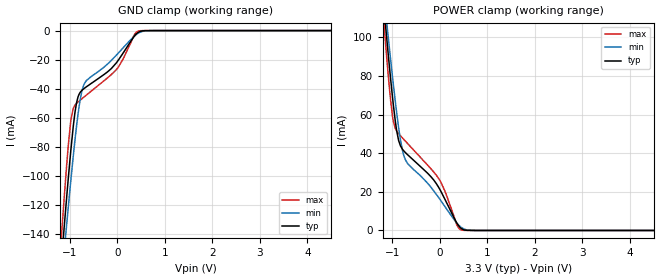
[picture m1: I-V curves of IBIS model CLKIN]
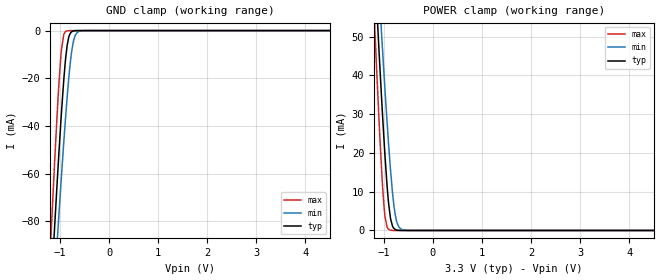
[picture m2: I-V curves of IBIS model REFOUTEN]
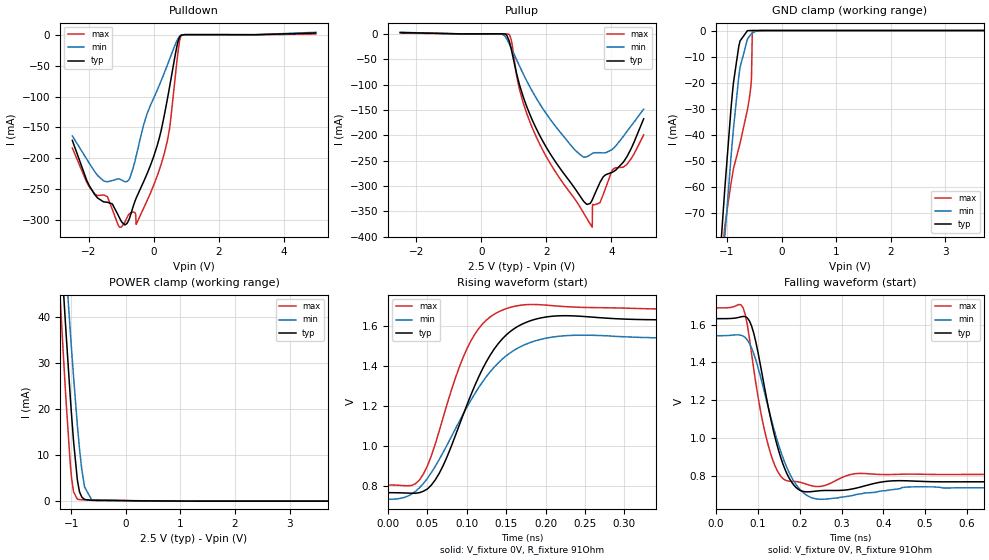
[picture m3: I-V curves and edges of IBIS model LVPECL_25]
| Texas Instruments Incorporated
| 3-GHz, 8-Output Differential Fanout Buffer / Level Translator
| Marketing part#   Voltage Range   Package-type   #pins/pkg drawing
| LMK00338   3.15V - 3.45V   LLP   40-pin SQ
[IBIS Ver]   4.1
[File name]   lmk00338.ibs
[File Rev]   1.1
[Date]   1/27/2014
[Source]   Model built from spectre simulations at:
   Texas Instruments Incorporated.
   Analog-eLab, HPA
   12500 TI Blvd
   Dallas, TX -75243
   For Support e-mail: elab_ibis@list.ti.com
[Notes]   Revision History
   Rev 1.1: 1/27/2014
   - Correct pin names/assignments for Pins 11, 19 and 32
   Rev 1.0: 3/12/2012
   - ccomp values are based on PVT settings:
   WEAK: Low Voltage, High Temperature, Weak Process
   NOM: Nominal Voltage, Nominal Temperature, Nominal Process
   STRONG: High Voltage, Low Temperature, Fast Process
   - User may change ccomp in the order of number values as
   per end simulator used
   - C_comp although listed in numberical order of value are obtained from varying PVT conditions.
   For PVT conditions for eachspecific value, refer to the buffer description under repective [Model].
   IBIS model user is responsible for using appropriate C_comp to simulate for Signal Integrity.
   - LVPECL Simulation recommendation:
   Use low value (1nF or less) for AC coupling.
   Larger values will result in long settling times.
   -PullUp and Pulldown non-monotonic for LVPECL and REFOUT models
[Disclaimer]  This model is designed as an aid for customers of Texas Instruments
 TI and its licensors and suppliers make no warranties, either expressed
 or implied, with respect to this  model, including the warranties of
 merchantability or fitness for a particular purpose.
 The model is provided solely on an "as is" basis. The entire risk as to
 its quality and performance is with the customer.
[Copyright] (C)Copyright 2012 Texas Instruments Incorporated.
   All rights reserved.
[Component]   LMK00308SQ
[Manufacturer]  Texas Instruments Incorporated
[Package]   |40-pin LLP SQ package
|   typ   min   max
R_pkg   0   0   0
L_pkg   0   0   0
C_pkg   0   0   0
[Pin]   signal_name   model_name   R_pin   L_pin   C_pin
1   CLKoutA0   DIFFOUT
2   CLKoutA0*   DIFFOUT
3   VCC0A   POWER
4   CLKoutA1   DIFFOUT
5   CLKoutA1*   DIFFOUT
6   VCC0A   POWER
7   CLKoutA2   DIFFOUT
8   CLKoutA2*   DIFFOUT
9   CLKout32   DIFFOUT
10   CLKout32*   DIFFOUT
11   CLKoutA_EN   REFOUTEN
12   VCC   POWER
13   OSCin   NC
14   OSCout   NC
15   CLKin_SEL0   NC
16   CLKin0   CLKIN
17   CLKin0*   CLKIN
18   CLKin_SEL1   NC
19   CLKoutB_EN   REFOUTEN
20   GND   GND
21   CLKoutB3*   DIFFOUT
22   CLKoutB3   DIFFOUT
23   CLKoutB2*   DIFFOUT
24   CLKoutB2   DIFFOUT
25   VCC0B   POWER
26   CLKoutB1*   DIFFOUT
27   CLKoutB1   DIFFOUT
28   VCC0B   POWER
29   CLKoutB0*   DIFFOUT
30   CLKoutB0   DIFFOUT
31   GND   GND
32   VCC   POWER
33   CLKin1*   CLKIN
34   CLKin1   CLKIN
35   VCC   POWER
36   REFout   REFOUT
37   VCC0C   POWER
38   REFout_EN   REFOUTEN
39   CLKoutA_TYPE1   NC
40   GND   GND
41   DAP   NC
[Diff pin]  inv_pin  vdiff  tdelay_typ  tdelay_min  tdelay_max
 3   4   NA   0.0s   0.0s   0.0s
 6   7   NA   0.0s   0.0s   0.0s
 8   9   NA   0.0s   0.0s   0.0s
20   21   NA   0.0s   0.0s   0.0s
22   23   NA   0.0s   0.0s   0.0s
25   26   NA   0.0s   0.0s   0.0s
15   16   0.15   NA  NA  NA   | Diff-in
31   30   0.15   NA  NA  NA   | Diff-in
| Model REFOUT
[Model Selector]   REFOUT
REFOUT_33   3.3 volt Vcc
REFOUT_25   2.5 volt Vcc
| Model DIFFOUT
[Model Selector]   DIFFOUT
LVPECL_33   3.3 volt Vcc
LVPECL_25   2.5 volt Vcc
LVDS_33   3.3 volt Vcc
LVDS_25   2.5 volt Vcc
HCSL_33   3.3 volt Vcc
HCSL_25   2.5 volt Vcc
[Define Package Model]  llp40_lmk00308
[Manufacturer]  Unknown
[OEM]  Unknown
[Description]  ]  Evaled at 2GHz using Buildsheet AD#LMK00308SQ-01 RevA
[Number Of Pins]  41
[Pin Numbers]
|Pin Num   Terminal Name
1   | L1:1
2   | L2:2
3   | L3:3
4   | L4:4
5   | L5:5
6   | L6:6
7   | L7:7
8   | L8:8
9   | L9:9
10   | L10:10
11   | L11:11
12   | L12:12
13   | L13:13
14   | L14:14
15   | L15:15
16   | L16:16
17   | L17:17
18   | L18:18
19   | L19:19
20   | L20:20
21   | L21:21
22   | L22:22
23   | L23:23
24   | L24:24
25   | L25:25
26   | L26:26
27   | L27:27
28   | L28:28
29   | L29:29
30   | L30:30
31   | L31:31
32   | L32:32
33   | L33:33
34   | L34:34
35   | L35:35
36   | L36:36
37   | L37:37
38   | L38:38
39   | L39:39
40   | L40:40
41   | LDAP:41
[Model Data]
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[End Model Data]
[End Package Model]
| Models and submodels in the file (10): CLKIN (Input), REFOUTEN (Input), LVPECL_25 (3-state), LVPECL_33 (3-state), LVDS_25 (Output), LVDS_33 (Output), HCSL_25 (Open_source), HCSL_33 (Open_source), REFOUT_25 (Output), REFOUT_33 (Output)
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|   Model   CLKIN
[Model]   CLKIN
Model_type   Input
Vinl = 1.2
Vinh = 1.35
|   typ   min   max
C_comp   0.334pF   0.334pF   0.334pF
[Voltage Range]   3.3   3.125   3.465
[Temperature Range]   45   125   -40
[Power Clamp Reference]   3.3   3.125   3.465
[GND Clamp Reference]   0   0   0
[GND Clamp]
|   Voltage   I(typ)   I(min)   I(max)
-3.3V     -1.09A     -1.005A    -1.209A
-1.181V   -161.9mA   -176mA     -145.1mA
-1.112V   -133.8mA   -150.7mA   -113.6mA
-1.063V   -114.4mA   -133.1mA   -92.33mA
-973.5mV  -81.6mA    -102.3mA   -61.43mA
-924mV    -65.73mA   -86.12mA   -53.42mA
-854.7mV  -49.53mA   -65.42mA   -49.97mA
-775.5mV  -42.3mA    -46.78mA   -47.7mA
-706.2mV  -40.03mA   -37.67mA   -45.84mA
-3.3mV    -21.51mA   -16.37mA   -26.2mA
432.3mV   -1.452mA   -2.001mA   -480.3uA
6.59V     0A         0A         0A
[POWER Clamp]
|   Voltage   I(typ)   I(min)   I(max)
-3.3V     736.4mA    674.5mA    821.9mA
-1.181V   117.5mA    123.8mA    109.8mA
-1.112V   98.9mA     107.1mA    88.87mA
-1.033V   78.62mA    88.59mA    67.5mA
-973.5mV  64.71mA    75.26mA    56.32mA
-914.1mV  53.13mA    62.75mA    51.87mA
-864.6mV  46.64mA    53.33mA    50.15mA
-745.8mV  40.96mA    38.12mA    46.9mA
-13.2mV   21.94mA    16.71mA    26.59mA
353.1mV   4.136mA    4.038mA    3.278mA
442.2mV   1.233mA    1.8mA      362.3uA
6.59V     0A         0A         0A
|   Model REFOUTEN
[Model]   REFOUTEN
Model_type   Input
Vinl = 0.8
Vinh = 2.0
|   typ   min   max
C_comp   0.3093pF   0.3093pF   0.3093pF
[Voltage Range]   3.3   3.125   3.465
[Temperature Range]   45   125   -40
[Power Clamp Reference]   3.3   3.125   3.465
[GND Clamp Reference]   0   0   0
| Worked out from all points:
|   GND clamp passes 1 mA (typ) near -0.79 V on its own axis
|   POWER clamp passes 1 mA (typ) near -0.82 V on its own axis
[GND Clamp]
|   Voltage   I(typ)   I(min)   I(max)
-3.3V     -965.6mA   -893.6mA   -1.069A
-1.181V   -108.3mA   -129.3mA   -84.35mA
-1.112V   -82.59mA   -106mA     -55.39mA
-1.043V   -57.82mA   -83.32mA   -28.72mA
-973.5mV  -34.81mA   -61.42mA   -8.124mA
-924mV    -20.4mA    -46.56mA   -1.597mA
-884.4mV  -11.09mA   -35.36mA   -347uA
-825mV    -2.889mA   -20.4mA    -26.1uA
-745.8mV  -310.8uA   -6.404mA   -528.4nA
-676.5mV  -33.31uA   -1.499mA   -14.52nA
-577.5mV  -943.1nA   -148.2uA   0A
6.59V     0A         0A         0A
[POWER Clamp]
|   Voltage   I(typ)   I(min)   I(max)
-3.3V     638.8mA    590.5mA    708.3mA
-1.191V   69.15mA    82.63mA    53.96mA
-1.181V   66.68mA    80.4mA     51.15mA
-1.102V   47.28mA    62.82mA    29.5mA
-1.033V   31.21mA    47.91mA    12.87mA
-993.3mV  22.67mA    39.68mA    5.73mA
-933.9mV  11.5mA     27.94mA    888.7uA
-864.6mV  3.112mA    15.73mA    67.37uA
-805.2mV  711.5uA    7.563mA    4.089uA
-745.8mV  145.3uA    2.701mA    212.4nA
-577.5mV  412.5nA    72uA       0A
6.59V     0A         0A         0A
|   Model LVPECL_25
[Model]   LVPECL_25
Model_type   3-state
Polarity   Non-Inverting
Rref =   91.0000
Vmeas =   1.99
|   typ   min   max
|   Nom   Strong   Weak
C_comp   2.0749pF   1.9512pF   2.2734pF
|Output in low   Nom   Strong   Weak
|C_Comp   2.0749pF   1.9512pF   2.2734pF
|Output in High   Nom   Strong   Weak
|C_Comp   0.7651pF   0.6976pF   0.7651pF
[Voltage Range]   2.5   2.375   2.625
[Temperature Range]   45   125   -40
[Pullup Reference]   2.5   2.375   2.625
[Pulldown Reference]   -0   0   -0
[Power Clamp Reference]   2.5   2.375   2.625
[GND Clamp Reference]   0   -0   -0
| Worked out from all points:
|   slope of the pulldown table from 0 to 0.375 V, typ, clamps not added: 4.73 ohm
|   GND clamp passes 1 mA (typ) near -0.66 V on its own axis
|   POWER clamp passes 1 mA (typ) near -0.81 V on its own axis
|   falling waveform, V_fixture 0V, R_fixture 91Ohm: 20-80 % time 48.8ps typ, 60.3ps min, 41.4ps max; typ from 1.63 V to 0.768 V
|   rising waveform, V_fixture 0V, R_fixture 91Ohm: 20-80 % time 56ps typ, 71.7ps min, 45.7ps max; typ from 0.768 V to 1.63 V
[Pulldown]
|   Voltage   I(typ)   I(min)   I(max)
-2.5V     -170.9mA   -163.7mA   -183.2mA
-1.817V   -258mA     -220.8mA   -256.9mA
-1.42V    -270.8mA   -237.8mA   -261.8mA
-1.045V   -296.5mA   -233.4mA   -311.1mA
-880mV    -307.5mA   -237.7mA   -302.8mA
-625mV    -277.3mA   -215.2mA   -286.5mA
-535mV    -264.3mA   -196.5mA   -306.6mA
-205mV    -225.5mA   -128.7mA   -269.1mA
245mV     -152.3mA   -73.16mA   -207.5mA
492.5mV   -84.88mA   -39.88mA   -152mA
845mV     -1.078mA   -1.179mA   -2.211mA
4.992V    2.59mA     3.71mA     981.9uA
[GND Clamp]
|   Voltage   I(typ)   I(min)   I(max)
-2.5V     -680.7mA   -652.3mA   -694.7mA
-1.135V   -89.97mA   -107.4mA   -101.7mA
-1.045V   -62.74mA   -81.12mA   -76.76mA
-1.038V   -60.54mA   -78.99mA   -75.08mA
-925mV    -30mA      -48.72mA   -58.7mA
-880mV    -20.04mA   -37.72mA   -53.1mA
-760mV    -4.036mA   -14.22mA   -43.38mA
-625mV    -70.9uA    -3.386mA   -30.51mA
-572.5mV  -12.45uA   -1.77mA    -23.42mA
-550mV    -6.1uA     -1.283mA   -18.23mA
-535mV    -3.82uA    -1.017mA   0A
4.992V    0A         0A         0A
[Pullup]
|   Voltage   I(typ)   I(min)   I(max)
-2.5V     2.519mA    2.915mA    1.456mA
845mV     -12.71mA   -18.28mA   -985.4uA
1.167V    -99.82mA   -63.09mA   -109mA
1.58V     -172.3mA   -115.1mA   -187.8mA
2.84V     -301.8mA   -226.4mA   -322.9mA
3.245V    -336.5mA   -242.4mA   -364.4mA
3.41V     -327.6mA   -236.1mA   -381.3mA
3.417V    -326.6mA   -235.8mA   -336.4mA
3.65V     -292.8mA   -234.5mA   -332.6mA
4.032V    -272.8mA   -227.6mA   -268.4mA
4.475V    -242.6mA   -192.8mA   -257.7mA
4.992V    -167.7mA   -148.6mA   -199.2mA
[POWER Clamp]
|   Voltage   I(typ)   I(min)   I(max)
-2.5V     367mA      361.7mA    377.1mA
-1.21V    59.59mA    72.33mA    46.61mA
-1.143V   46.29mA    59.65mA    32.09mA
-1.105V   39.1mA     52.81mA    24.38mA
-1.09V    36.27mA    50.11mA    21.4mA
-1.015V   22.74mA    37.01mA    8.205mA
-955mV    13.09mA    27.12mA    2.027mA
-880mV    4.226mA    15.88mA    429.9uA
-805mV    886.5uA    6.959mA    296.1uA
-752.5mV  360.6uA    3.052mA    282.5uA
-595mV    172.5uA    235uA      254.5uA
4.992V    0A         0A         0A
[Ramp]
R_load = 91
|   typ   min   max
dV/dt_r   0.518031/5.60422e-11   0.48219/7.16356e-11   0.529005/4.56696e-11
dV/dt_f   0.518044/4.88422e-11   0.482317/6.01916e-11   0.528924/4.14467e-11
[Falling Waveform]
V_fixture = 0V
V_fixture_min = 0V
V_fixture_max = 0V
R_fixture = 91Ohm
C_fixture = 0F
|   Time   V(typ)   V(min)   V(max)
0s        1.631V     1.541V     1.688V
60ps      1.641V     1.543V     1.704V
80ps      1.619V     1.5V       1.526V
105ps     1.399V     1.335V     1.16V
125ps     1.163V     1.16V      960mV
170ps     808mV      839.7mV    772.7mV
200ps     723.2mV    729.1mV    765.5mV
250ps     720.4mV    674.6mV    743.2mV
340ps     736.6mV    701.6mV    811.6mV
1.39ns    767.8mV    735.5mV    806.5mV
[Rising Waveform]
V_fixture = 0V
V_fixture_min = 0V
V_fixture_max = 0V
R_fixture = 91Ohm
C_fixture = 0F
|   Time   V(typ)   V(min)   V(max)
0s        767.7mV    734.5mV    806.3mV
35ps      764.9mV    775mV      813mV
55ps      805.9mV    868.2mV    952.3mV
85ps      1.048V     1.083V     1.335V
105ps     1.255V     1.229V     1.526V
135ps     1.487V     1.396V     1.661V
165ps     1.6V       1.491V     1.703V
200ps     1.646V     1.54V      1.706V
245ps     1.649V     1.555V     1.694V
1.38ns    1.631V     1.539V     1.688V
